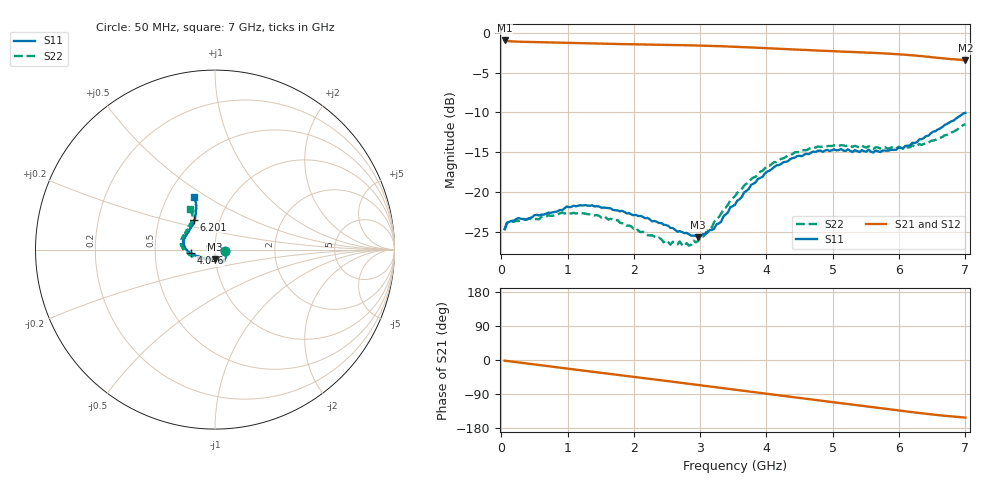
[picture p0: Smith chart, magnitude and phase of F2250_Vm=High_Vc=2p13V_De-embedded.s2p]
! Integrated Device Technology
! Corporate Headquarters
! 6024 Silver Creek Valley Road
! San Jose, CA 95138  USA
! Phone:  1-408-284-8200
! Toll Free:  1-800-223-1366
! Webpage:  http://www.idt.com/
! Timing and RF Division
! 515 Groton Road, Suite 102
! Westford, MA 01886-6024
! Device:  F2250
! Description: Voltage Variable RF Attenuator
! Frequency:  50.0 -  6000.00 MHz
! Package:  3x3 mm Thin QFN Plastic Package: 16 pin
! Ports:  2 RF, 3 DC
!  Pin  1  = GND
!  Pin  2  = NC
!  Pin  3  = RF1  = Port 1
!  Pin  4  = NC
!  Pin  5  = GND
!  Pin  6  = GND
!  Pin  7  = GND
!  Pin  8  = GND
!  Pin  9  = NC
!  Pin 10  = RF2  = Port 2
!  Pin 11  = NC
!  Pin 12  = GND
!  Pin 13  = GND
!  Pin 14  = VCNTRL
!  Pin 15  = VDD
!  Pin 16  = VMODE
! Vcntrl:  2.130 Volts
! Vmode:  +3.300 Volts
! Vdd:  +3.30  Volts
! Current:  1.319 mA
! Data:  The device was measured on a the F2250 evaluation board which has
!  individual transmission lines to the RF pins.  Data was collected
!  using a calibrated network analyzer.  The evaluation board was
!  de-embedded using a TRL calibration technique.
!  The reference plane is the edge of the package pin.
! Misc:  SN 10
!  Action Tracker AT0258
! Date Measured:  2014-11-26
! Date:  2015-10-15  MJV
! Note:
!  Integrated Device Technology supplies this data as a sample of measured
!  data at the package pin for this product.  Your particular data for this
!  product may vary.
!  Data was taken at 25 degrees C.
!  Integrated Device Technology reserves the right to change this data at anytime.
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# GHz S dB R 50
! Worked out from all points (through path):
!   201 points, 50 MHz to 7 GHz, reference 50 ohm
!   highest |S21| = -0.95 dB at 50 MHz (marker M1); lowest = -3.4 dB at 7 GHz (marker M2)
!   group delay of S21, straight-line fit = 61.1 ps
!   lowest |S11| = -25.7 dB at 2.969 GHz (marker M3), VSWR 1.11, Z = 49.6 - j5.16 ohm
!   |S11| at or under -10 dB: start of sweep to end of sweep
!   |S22| runs from -26.8 to -11.5 dB; largest |S21 - S12| = 0.0019
!   S11 on the Smith chart (normalised r, x): 50 MHz: 1.12, -0.02; 4.046 GHz: 0.76, -0.03; 6.201 GHz: 0.75, +0.26; 7 GHz: 0.68, +0.44
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0.05  -24.66 -9.6  -0.95 -1.8  -0.95 -1.8  -24.86 -10.0
0.08475  -23.89 -8.7  -1.02 -2.5  -1.02 -2.5  -23.95 -8.9
0.1195  -23.77 -9.3  -1.05 -3.3  -1.05 -3.2  -23.76 -8.4
0.91875  -22.30 -47.0  -1.24 -21.0  -1.24 -21.1  -22.59 -49.1
1.2315  -21.73 -54.7  -1.31 -27.9  -1.31 -27.9  -22.71 -59.6
1.75275  -22.34 -61.6  -1.40 -39.1  -1.40 -39.1  -23.55 -66.8
2.37825  -23.93 -61.8  -1.49 -52.8  -1.49 -52.8  -25.77 -68.4
2.552  -24.54 -66.3  -1.51 -56.6  -1.51 -56.6  -26.64 -74.9
2.691  -24.96 -73.6  -1.54 -59.7  -1.54 -59.7  -26.25 -82.2
2.7605  -25.19 -75.6  -1.55 -61.3  -1.55 -61.3  -26.84 -86.5
2.969  -25.68 -92.0  -1.59 -66.0  -1.59 -66.0  -26.19 -104.6
3.21225  -24.61 -121.5  -1.65 -71.4  -1.65 -71.5  -23.77 -128.6
3.525  -21.62 -148.1  -1.74 -78.5  -1.74 -78.5  -20.55 -147.3
3.76825  -19.12 -161.4  -1.84 -84.0  -1.84 -84.0  -18.39 -158.5
4.04625  -17.34 -171.4  -1.95 -90.2  -1.95 -90.2  -16.72 -169.0
4.4285  -15.71 178.1  -2.09 -98.6  -2.10 -98.6  -15.02 179.5
4.7065  -14.93 171.0  -2.19 -104.8  -2.20 -104.8  -14.52 173.6
5.054  -14.78 162.8  -2.32 -112.4  -2.32 -112.5  -14.13 166.4
5.85325  -14.79 136.7  -2.62 -130.0  -2.62 -130.1  -14.54 147.6
6.20075  -13.84 124.8  -2.83 -137.7  -2.83 -137.8  -14.13 138.5
6.54825  -12.38 116.6  -3.10 -144.7  -3.10 -144.8  -13.48 127.1
7  -10.06 111.6  -3.43 -152.0  -3.44 -152.2  -11.48 120.8
